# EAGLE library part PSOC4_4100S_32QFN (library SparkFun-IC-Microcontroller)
PSOC4100 CY8C4146LQI-S422 PSOC4100S 64k FLASH, 8K RAM, 32QFN SparkFun Products SparkFun Serial Controlled Motor Driver
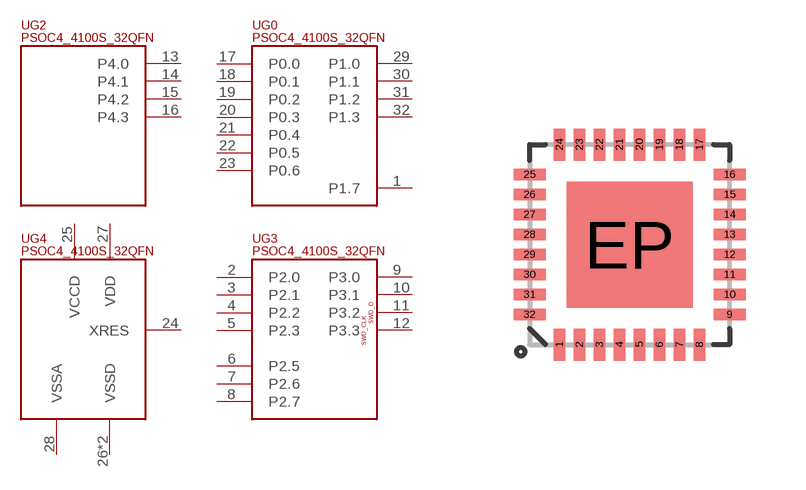
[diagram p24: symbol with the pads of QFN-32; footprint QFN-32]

Designator prefix U; gates G2=PSOC_4100S_32QFN_PORT_4 G0=PSOC_4100S_32QFN_PORTS_0_AND_1 G3=PSOC_4100S_32QFN_PORTS_2_AND_3 G4=PSOC_4100S_QFN32_POWER

## PSOC4_4100S_32QFN (PROD_ID: IC-13286; VALUE: CY8C4146LQI-S422)  [QFN-32]
1  G0:P1.7
2  G3:P2.0
3  G3:P2.1
4  G3:P2.2
5  G3:P2.3
6  G3:P2.5
7  G3:P2.6
8  G3:P2.7
9  G3:P3.0
10  G3:P3.1
11  G3:P3.2
12  G3:P3.3
13  G2:P4.0
14  G2:P4.1
15  G2:P4.2
16  G2:P4.3
17  G0:P0.0
18  G0:P0.1
19  G0:P0.2
20  G0:P0.3
21  G0:P0.4
22  G0:P0.5
23  G0:P0.6
24  G4:XRES
25  G4:VCCD
26  G4:VSSD
27  G4:VDD
28  G4:VSSA
29  G0:P1.0
30  G0:P1.1
31  G0:P1.2
32  G0:P1.3
EP  G4:VSSD

## Footprint QFN-32 (pad centres in mm)
QFN 32-Pin package w/ Thermal Pad ***Unproven*** Applicable Parts: TLC5940
smd 0.285 x 0.8: 1 -1.75,-2.5; 2 -1.25,-2.5; 3 -0.75,-2.5; 4 -0.25,-2.5; 5 0.25,-2.5; 6 0.75,-2.5; 7 1.25,-2.5; 8 1.75,-2.5; 17 1.75,2.5; 18 1.25,2.5; 19 0.75,2.5; 20 0.25,2.5; 21 -0.25,2.5; 22 -0.75,2.5; 23 -1.25,2.5; 24 -1.75,2.5
smd 0.8 x 0.285: 9 2.5,-1.75; 10 2.5,-1.25; 11 2.5,-0.75; 12 2.5,-0.25; 13 2.5,0.25; 14 2.5,0.75; 15 2.5,1.25; 16 2.5,1.75; 25 -2.5,1.75; 26 -2.5,1.25; 27 -2.5,0.75; 28 -2.5,0.25; 29 -2.5,-0.25; 30 -2.5,-0.75; 31 -2.5,-1.25; 32 -2.5,-1.75
smd 3.15 x 3.15: EP 0,0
